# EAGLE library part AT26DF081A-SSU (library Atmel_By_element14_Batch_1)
8-megabit 2.7-volt Minimum SPI Serial Flash Memory
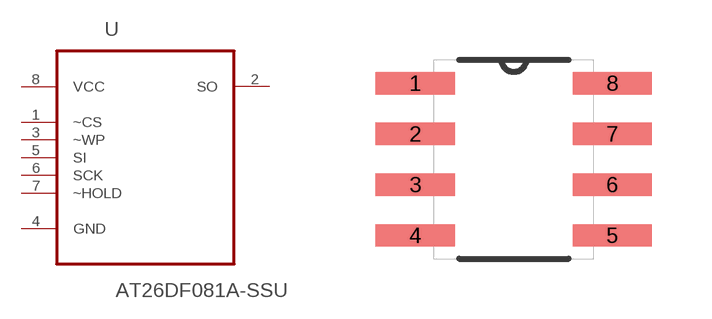
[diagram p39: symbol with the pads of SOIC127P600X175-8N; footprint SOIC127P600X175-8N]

Designator prefix U

## AT26DF081A-SSU (MPN: AT26DF081A-SSU; OC_FARNELL: 1715448; OC_NEWARK: -; PACKAGE: SOIC-8; SUPPLIER: Atmel)  [SOIC127P600X175-8N]
1  ~CS  in
2  SO  out
3  ~WP  in
4  GND  pas
5  SI  in
6  SCK  in
7  ~HOLD  in
8  VCC  pwr

## Footprint SOIC127P600X175-8N (pad centres in mm)
smd 1.981 x 0.559: 1 -2.464,1.905; 2 -2.464,0.635; 3 -2.464,-0.635; 4 -2.464,-1.905; 5 2.464,-1.905; 6 2.464,-0.635; 7 2.464,0.635; 8 2.464,1.905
